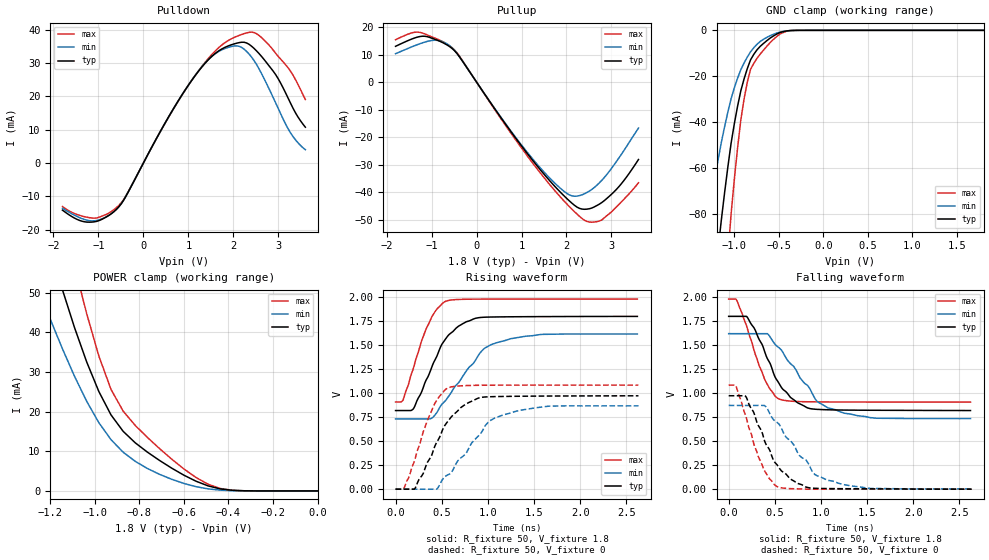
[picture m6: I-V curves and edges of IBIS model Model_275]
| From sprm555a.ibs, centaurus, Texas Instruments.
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| Model based on original model for BCSHTLTCSCDDVPBFZ_SSGFV
|   Sub model SR11_9MA_PADP_10PER_1P8
[model]   Model_275
|[Description]  [1.8V-3-STATE-X-SLOWEST:9MA, IND, 10%]
|   Slowest slew rate (SR[1:0] = "11"), 0.88 * RExt = 1.125 * Iout
|   (I[2:0] = "100"), 9mA nominal with Rext = 50R, ,Industrial
|   temperature range (-40C to 125C, 25C nominal),10% power supply
|   tolerance
|[Input Load]
|[Output Drive] SLOWEST:9MA
|Voltage   1.8V
|Mode   3-STATE
Model_type   3-state
Polarity   Non-Inverting
Enable   Active-Low
Cref =  15pF
Rref =  100.0000M
Vref =  0V
Vmeas =  0.9
C_comp   1.851324p   1.663768p   1.973575p
[Temperature Range]   25   125   -40
[Voltage Range]   1.8   1.62   1.98
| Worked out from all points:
|   slope of the pulldown table from 0 to 0.27 V, typ, clamps not added: 39.3 ohm
|   slope of the pullup table from 0 to 0.27 V, typ, clamps not added: 41.3 ohm
|   GND clamp passes 1 mA (typ) near -0.49 V on its own axis
|   POWER clamp passes 1 mA (typ) near -0.47 V on its own axis
|   rising waveform, R_fixture 50, V_fixture 1.8: 20-80 % time 290ps typ, 407ps min, 230ps max; typ from 0.819 V to 1.8 V
|   rising waveform, R_fixture 50, V_fixture 0: 20-80 % time 319ps typ, 397ps min, 239ps max; typ from 0 V to 0.972 V
|   falling waveform, R_fixture 50, V_fixture 1.8: 20-80 % time 310ps typ, 386ps min, 233ps max; typ from 1.8 V to 0.819 V
|   falling waveform, R_fixture 50, V_fixture 0: 20-80 % time 289ps typ, 394ps min, 227ps max; typ from 0.973 V to 0 V
[POWER_clamp]
-1.8V     194.9mA    137.1mA    262.8mA
-1.236V   68.49mA    48.51mA    92.67mA
-1.145V   50.76mA    35.86mA    69.65mA
-1.127V   47.56mA    33.54mA    65.34mA
-1.055V   35.4mA     24.69mA    48.69mA
-981.8mV  25.06mA    17.2mA     34.01mA
-927.3mV  19.17mA    12.93mA    25.61mA
-872.7mV  15.03mA    9.767mA    20.12mA
-818.2mV  12.12mA    7.45mA     16.5mA
-654.5mV  5.738mA    2.93mA     8.003mA
-436.4mV  508.2uA    199.4uA    613uA
0V        2.273nA    15.95nA    16.67nA
[Pulldown]
-1.8V     -14.14mA   -13.59mA   -13.06mA
-1.145V   -17.74mA   -17.37mA   -16.51mA
-545.5mV  -13.15mA   -13.12mA   -12.71mA
545.5mV   13.5mA     13.52mA    13.41mA
1.091V    25.12mA    25.21mA    25.13mA
1.527V    32.11mA    32.07mA    32.67mA
1.964V    35.54mA    35.01mA    37.35mA
2.291V    36.06mA    33.55mA    39.05mA
2.618V    32.13mA    27.06mA    37.75mA
2.945V    26.42mA    17.9mA     32.85mA
3.218V    19.44mA    10.24mA    28.56mA
3.6V      10.76mA    3.999mA    19.09mA
[Pullup]
-1.8V     12.99mA    10.3mA     15.38mA
-1.2V     16.67mA    14.26mA    17.79mA
-872.7mV  15.21mA    15.17mA    15.62mA
-600mV    12.91mA    13.24mA    13.19mA
-381.8mV  9.242mA    9.222mA    9.473mA
1.2V      -27.49mA   -27.01mA   -28.42mA
1.745V    -38.03mA   -36.86mA   -39.59mA
2.127V    -44.16mA   -41.42mA   -46.35mA
2.455V    -46.24mA   -40.18mA   -50.71mA
2.727V    -44.44mA   -36.72mA   -50.57mA
3.164V    -38.07mA   -27.64mA   -44.53mA
3.6V      -28.19mA   -16.75mA   -36.64mA
[GND_clamp]
-1.8V     -346.1mA   -209.3mA   -568.3mA
-1.327V   -149.7mA   -89.03mA   -250.9mA
-1.291V   -135.6mA   -80.47mA   -227.5mA
-1.145V   -82.35mA   -48.67mA   -137.7mA
-1.073V   -59.44mA   -35.55mA   -97.96mA
-1.036V   -49.1mA    -29.72mA   -79.9mA
-927.3mV  -26.31mA   -17.11mA   -38.99mA
-854.5mV  -16.67mA   -11.64mA   -22.56mA
-818.2mV  -12.86mA   -9.351mA   -16.98mA
-672.7mV  -5.705mA   -3.913mA   -8.624mA
-381.8mV  -120.4uA   -129uA     -167.4uA
1.8V      2.273nA    454nA      6.646nA
[Ramp]
dV/dt_f 0.59100197/0.31184562n 0.53539496/0.38923992n 0.64489294/0.23437504n
dV/dt_r 0.58616018/0.32018107n  0.5265456/0.39861668n 0.65183721/0.23915426n
R_load = 50
[Rising Waveform]
R_fixture = 50
V_fixture = 1.8
V_fixture_min = 1.62
V_fixture_max = 1.98
0s        818.8mV    731.8mV    908.1mV
81ps      818.8mV    731.8mV    926.4mV
197.6ps   843.7mV    731.8mV    1.273V
285.5ps   1.02V      731.8mV    1.554V
390.5ps   1.266V     738.2mV    1.79V
543.5ps   1.567V     924.8mV    1.957V
766.8ps   1.744V     1.232V     1.978V
1.035ns   1.793V     1.505V     1.98V
1.569ns   1.797V     1.611V     1.98V
2.62ns    1.799V     1.616V     1.98V
[Rising Waveform]
R_fixture = 50
V_fixture = 0
V_fixture_min = 0
V_fixture_max = 0
0s        0V         0V         0V
85.6ps    0V         0V         0V
208.5ps   4.446mV    0V         304.2mV
410.4ps   406mV      0V         863.6mV
567ps     706.4mV    149.2mV    1.054V
792.5ps   902mV      424.2mV    1.08V
1.013ns   962.4mV    707mV      1.083V
1.121ns   964.9mV    757.1mV    1.083V
1.658ns   969.9mV    864.4mV    1.084V
2.632ns   972.3mV    867.7mV    1.084V
[Falling Waveform]
R_fixture = 50
V_fixture = 1.8
V_fixture_min = 1.62
V_fixture_max = 1.98
0s        1.799V     1.619V     1.979V
90.6ps    1.799V     1.619V     1.962V
204.9ps   1.786V     1.619V     1.665V
389.6ps   1.433V     1.619V     1.144V
548.8ps   1.096V     1.47V      937.7mV
758ps     893.6mV    1.186V     911.9mV
956.7ps   831mV      915.6mV    908.9mV
1.077ns   826.4mV    845.9mV    907.8mV
1.6ns     821.3mV    738.5mV    907.1mV
2.62ns    818.7mV    734.6mV    907.1mV
[Falling Waveform]
R_fixture = 50
V_fixture = 0
V_fixture_min = 0
V_fixture_max = 0
0s        972.5mV    872mV      1.083V
83.6ps    972.5mV    872mV      1.064V
182ps     968.9mV    872mV      773.8mV
380.4ps   529.8mV    872mV      206.8mV
526.7ps   250.9mV    692.9mV    26.09mV
740.9ps   62.95mV    390.9mV    3.512mV
934.3ps   9.181mV    152.6mV    0V
1.071ns   6.28mV     92.31mV    0V
1.533ns   3.384mV    8.061mV    0V
2.632ns   0V         3.197mV    0V
